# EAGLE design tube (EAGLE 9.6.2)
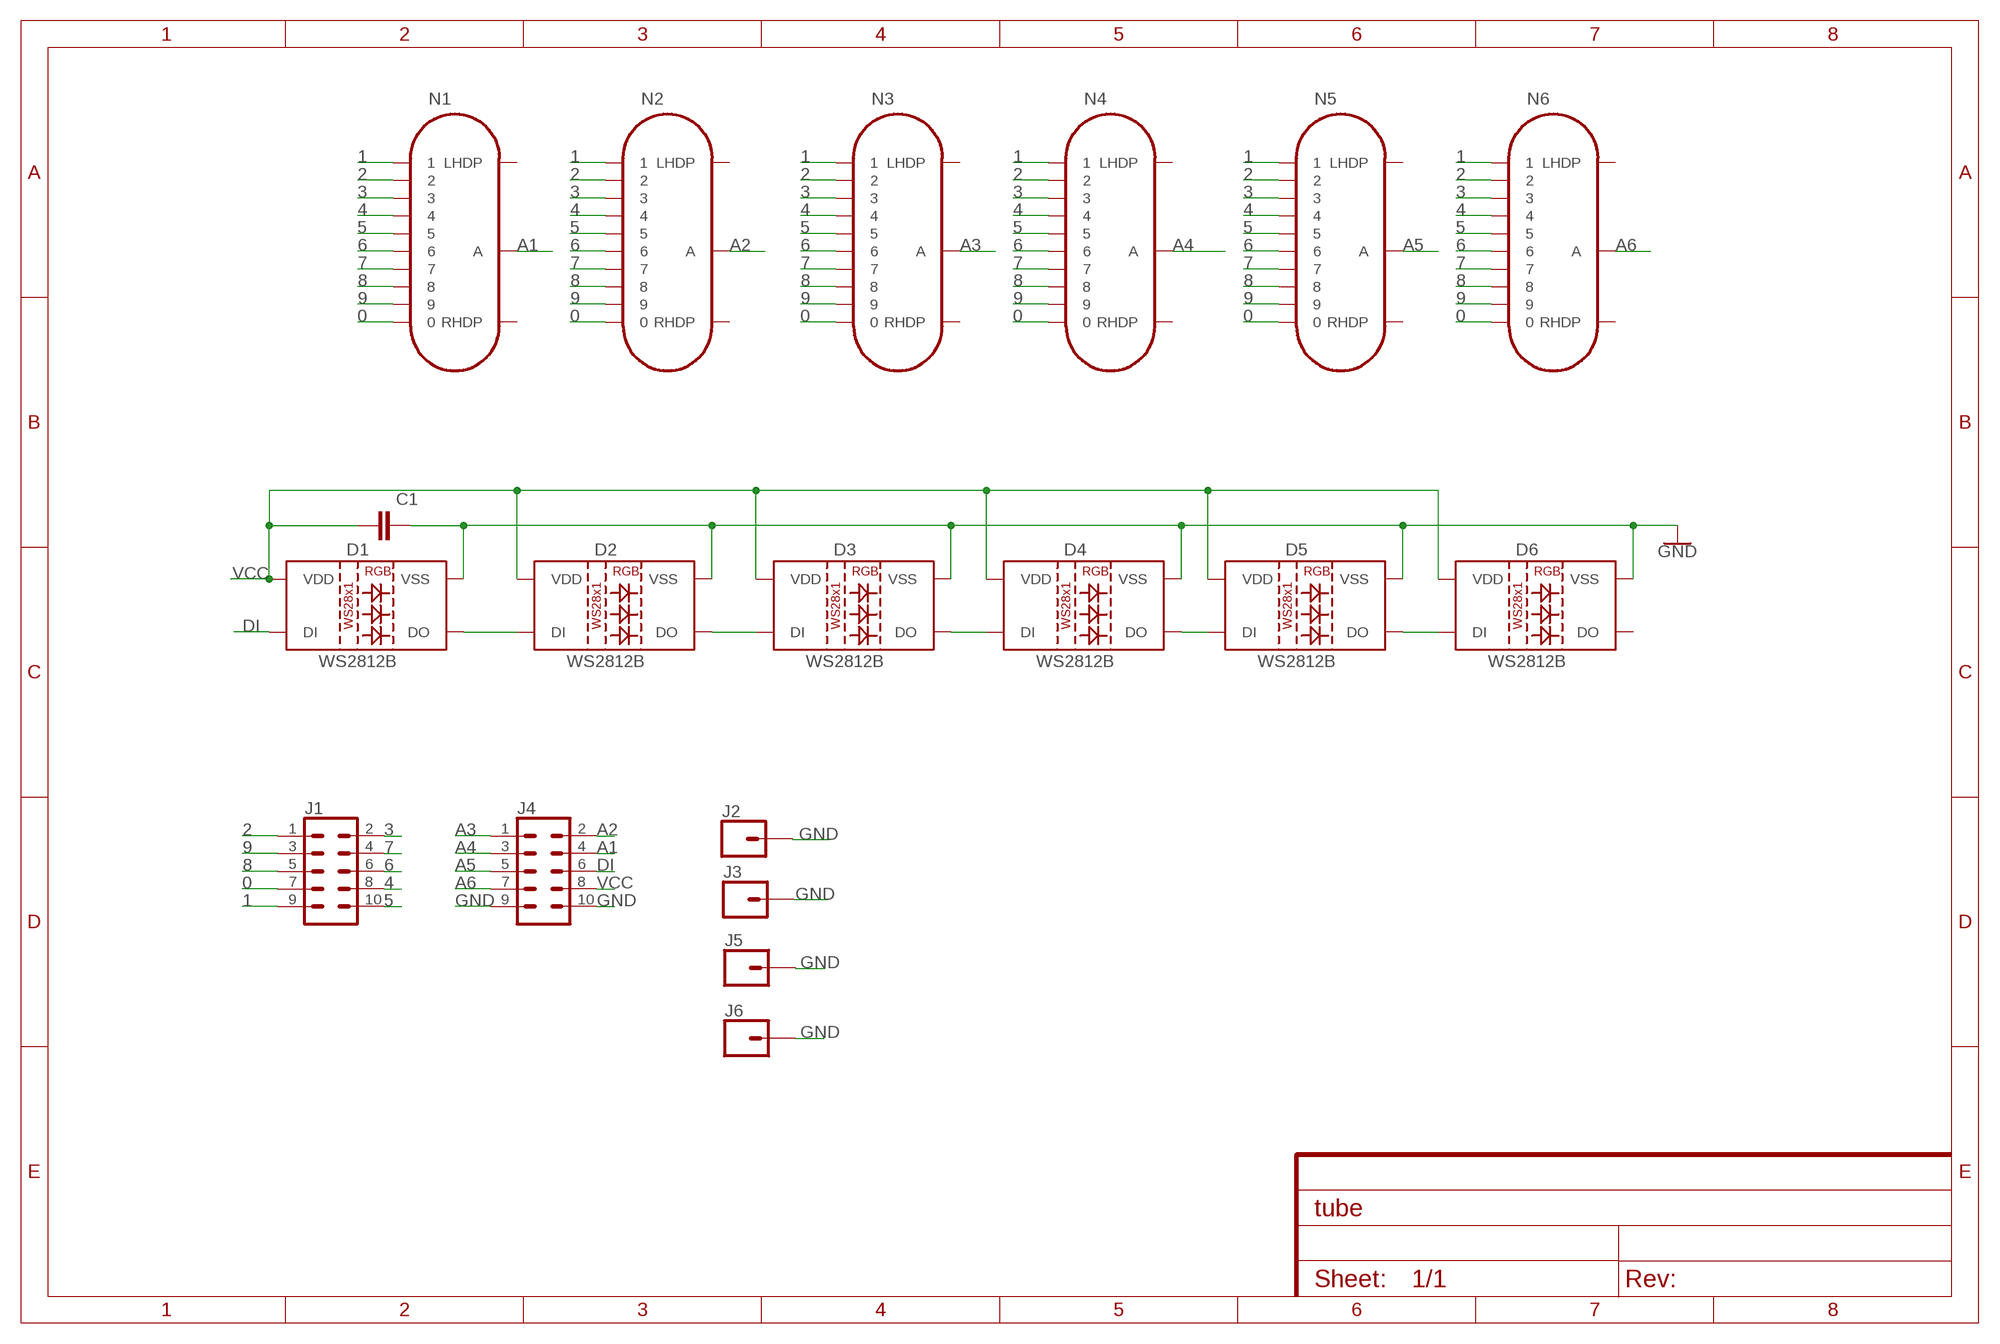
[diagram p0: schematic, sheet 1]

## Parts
C1  C-EUC1206  [C1206]
D1  WS2812B  [WS2812B]
D2  WS2812B  [WS2812B]
D3  WS2812B  [WS2812B]
D4  WS2812B  [WS2812B]
D5  WS2812B  [WS2812B]
D6  WS2812B  [WS2812B]
J1  CONN_05X2NO_SILK  [2X5_NOSILK]
J2  CONN_01PTH_2MM  [1X01_2MM]
J3  CONN_01PTH_2MM  [1X01_2MM]
J4  CONN_05X2NO_SILK  [2X5_NOSILK]
J5  CONN_01PTH_2MM  [1X01_2MM]
J6  CONN_01PTH_2MM  [1X01_2MM]
N1  IN-14  [IN-14]
N2  IN-14  [IN-14]
N3  IN-14  [IN-14]
N4  IN-14  [IN-14]
N5  IN-14  [IN-14]
N6  IN-14  [IN-14]

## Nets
0: J1.7 N1.0 N2.0 N3.0 N4.0 N5.0 N6.0
1: J1.9 N1.1 N2.1 N3.1 N4.1 N5.1 N6.1
2: J1.1 N1.2 N2.2 N3.2 N4.2 N5.2 N6.2
3: J1.2 N1.3 N2.3 N3.3 N4.3 N5.3 N6.3
4: J1.8 N1.4 N2.4 N3.4 N4.4 N5.4 N6.4
5: J1.10 N1.5 N2.5 N3.5 N4.5 N5.5 N6.5
6: J1.6 N1.6 N2.6 N3.6 N4.6 N5.6 N6.6
7: J1.4 N1.7 N2.7 N3.7 N4.7 N5.7 N6.7
8: J1.5 N1.8 N2.8 N3.8 N4.8 N5.8 N6.8
9: J1.3 N1.9 N2.9 N3.9 N4.9 N5.9 N6.9
A1: J4.4 N1.A
A2: J4.2 N2.A
A3: J4.1 N3.A
A4: J4.3 N4.A
A5: J4.5 N5.A
A6: J4.7 N6.A
DI: D1.4(DI) J4.6
GND: C1.2 D1.3(VSS) D2.3(VSS) D3.3(VSS) D4.3(VSS) D5.3(VSS) D6.3(VSS) J2.1 J3.1 J4.9 J4.10 J5.1 J6.1
N$1: D1.2(DO) D2.4(DI)
N$2: D2.2(DO) D3.4(DI)
N$3: D3.2(DO) D4.4(DI)
N$4: D4.2(DO) D5.4(DI)
N$5: D5.2(DO) D6.4(DI)
VCC: C1.1 D1.1(VDD) D2.1(VDD) D3.1(VDD) D4.1(VDD) D5.1(VDD) D6.1(VDD) J4.8
Unconnected: D6.2(DO) N1.LHDP N1.RHDP N2.LHDP N2.RHDP N3.LHDP N3.RHDP N4.LHDP N4.RHDP N5.LHDP N5.RHDP N6.LHDP N6.RHDP

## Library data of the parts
C1 = rcl:C-EU: CAPACITOR, European symbol; SPICEPREFIX: C
D1-D6 = SparkFun-LED:WS2812B: WS2812B SMD addressable RGB LED 5x5mm SMD LED with built-in controller IC. Color: Red/Green/Blue mC Rating: RGB: 390, 660, 180 mcd Forward Voltage: RGB: 2.0, 3.0, 3.0 V Packages:WS2812B SparkFun Products: Blynk Board - ESP8266; PROD_ID: DIO-12503
J1 J4 = SparkFun-Connectors:CONN_05X2: Multi connection point. Often used as Generic Header-pin footprint for 0.1 inch spaced/style header connections For AVR SPI programming port, see special device with nice symbol: "AVR_SPI_PROG_5x2.dev" You can populate with any combo of single row headers, but if you'd like an exact match, check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
J2 J3 J5 J6 = SparkFun-Connectors:CONN_01: Single connection point. Often used as Generic Header-pin footprint for 0.1 inch spaced/style header connections
N1-N6 = russian-nixies:IN-14: IN-14: medium numeric frontview nixie tube

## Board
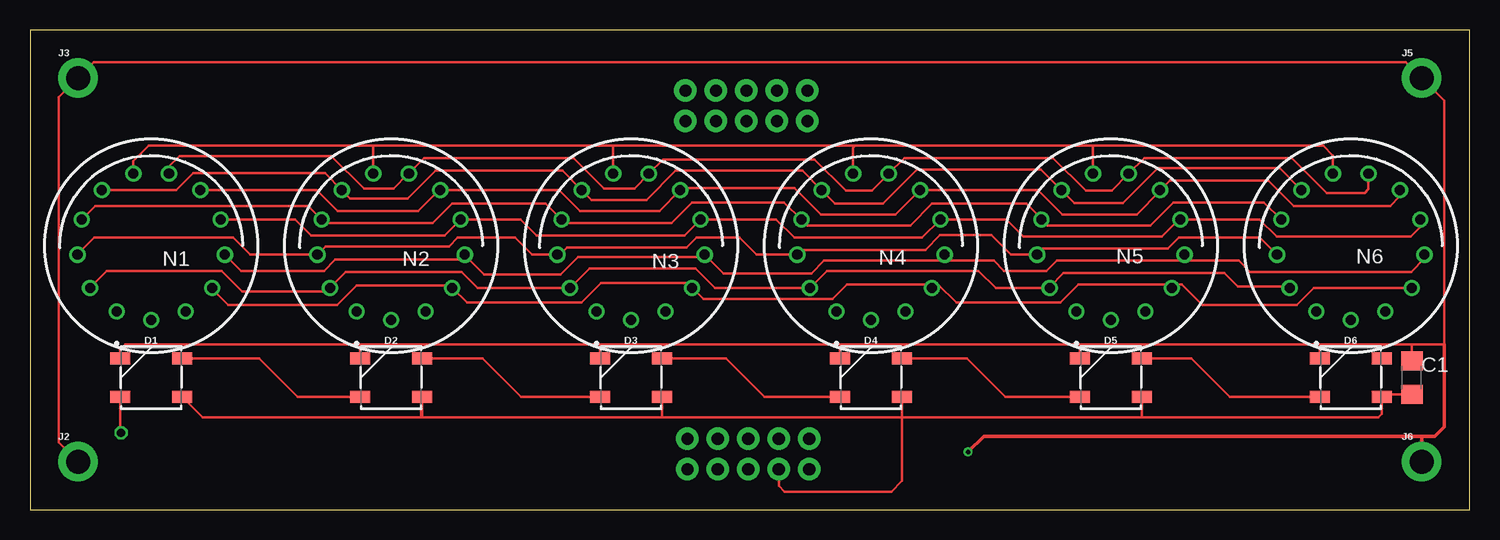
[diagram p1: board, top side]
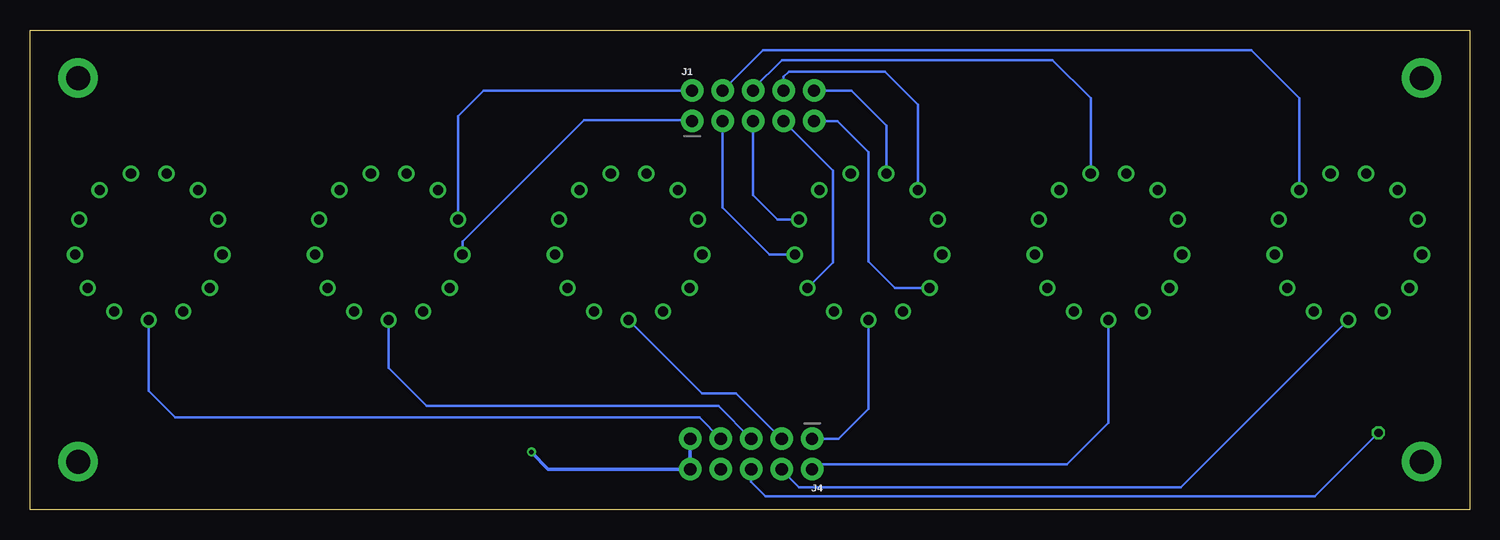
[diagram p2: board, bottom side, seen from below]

Size 120 x 40 mm. Coordinates in mm from the lower left corner, seen from the top.
Outline: 0,40 0,0 120,0 120,40 0,40
Copper layers (1*16): Top 0.035mm / dielectric 1.5mm / Bottom 0.035mm
Design rules "default": minimum track width 6mil, minimum drill 0.35mm, track to track 6mil, track to pad 6mil, pad to pad 6mil, via to via 6mil, smd to smd 6mil, copper to edge 40mil, drill to drill 6mil, minimum pad ring 10mil, minimum via ring 8mil, stop-mask expansion 4mil, vias tented up to drill 0mil, thermal gap 10mil

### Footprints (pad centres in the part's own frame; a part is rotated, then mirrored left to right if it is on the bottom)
C1206 = smd 1.6 x 1.8: 1 -1.4,0; 2 1.4,0
WS2812B = smd 1.651 x 1: 1 2.577,-1.6; 2 2.577,1.6; 3 -2.577,1.6; 4 -2.577,-1.6
2X5_NOSILK = drill 1.016 pad 1.88: 1 0,0; 2 0,2.54; 3 2.54,0; 4 2.54,2.54; 5 5.08,0; 6 5.08,2.54; 7 7.62,0; 8 7.62,2.54; 9 10.16,0; 10 10.16,2.54
1X01_2MM = drill 2 pad 3.302: 1 0,0
IN-14 = drill 0.84: 0 5.094,-3.516; 1 -5.094,-3.516; 2 -6.145,-0.746; 3 -5.788,2.195; 4 -4.105,4.633; 5 -1.481,6.01; 6 1.481,6.01; 7 4.105,4.633; 8 5.788,2.195; 9 6.145,-0.746; A 0,-6.19; LHDP 2.877,-5.481; RHDP -2.877,-5.481

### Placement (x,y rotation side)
C1  115.2,11 90 top
D1  10.1,11 0 top
D2  30.1,11 0 top
D3  50.1,11 0 top
D4  70.1,11 0 top
D5  90.1,11 0 top
D6  110.1,11 0 top
J1  64.8,32.4 0 bottom
J2  4,4 0 top
J3  4,36 0 top
J4  54.8,5.9 180 bottom
J5  116,36 0 top
J6  116,4 0 top
N1  10.1,22 0 top
N2  30.1,22 0 top
N3  50.1,22 0 top
N4  70.1,22 0 top
N5  90.1,22 0 top
N6  110.1,22 0 top

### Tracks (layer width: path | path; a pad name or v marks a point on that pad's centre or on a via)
0
  Top 0.2: N1.0 15.19,18.39 16.53,17.06 25.59,17.06 27.22,18.68 34.99,18.68 N2.0 35.21,18.48 36.43,17.26 45.99,17.26 47.62,18.88 54.79,18.88 N3.0 55.21,18.48 56.13,17.56 66.89,17.56 68.12,18.78 75.19,18.78 | 75.19,18.78 75.71,18.78 77.23,17.26 85.89,17.26 87.42,18.78 95.19,18.78 N5.0 95.19,18.68 95.29,18.78 96.01,18.78 97.73,17.06 105.59,17.06 107.02,18.48 N6.0 | N4.0 75.19,18.78
  Bottom 0.2: J1.7 53.06,28.28 53.06,20.61 N3.0
1
  Top 0.2: N1.1 5.01,18.5 6.41,19.91 15.98,19.91 17.71,18.18 24.71,18.18 N2.1 25.01,18.51 26.31,19.81 35.98,19.81 37.3,18.48 N3.1 46.64,20.11 55.48,20.11 57.1,18.48 N4.1 66.44,19.91 79.08,19.91 80.5,18.48 N5.1 85.01,18.57 86.14,19.71 99.58,19.71 100.7,18.58 104.91,18.58 N6.1
  Bottom 0.2: J1.9 52.7,32.4 50.1,29.8 50.1,20.7 47.88,18.48 N3.1
2
  Top 0.2: N1.2 3.96,21.27 5.36,22.68 16.93,22.68 18.36,21.25 N2.2 24.66,21.95 34.94,21.95 35.66,22.68 40.43,22.68 41.85,21.25 N3.2 44.16,21.25 44.76,21.85 54.73,21.85 55.56,22.68 59.13,22.68 60.55,21.25 N4.2 64.36,21.65 74.64,21.65 75.86,22.88 80.13,22.88 81.75,21.25 N5.2 84.45,21.75 94.83,21.75 95.76,22.68 102.53,22.68 N6.2 | N6.2
  Bottom 0.2: J1.1 64.9,32.5 73.81,32.5 83.95,22.35 N5.2
3
  Top 0.2: N1.3 5.44,25.32 23.19,25.32 N2.3 24.61,23.89 33.58,23.89 35.2,25.52 42.97,25.52 44.3,24.2 N3.3 44.61,23.89 53.48,23.89 55.2,25.62 62.87,25.62 64.3,24.2 N4.3 64.81,23.7 73.38,23.7 75.2,25.52 83.07,25.52 84.31,24.28 N5.3 84.81,23.7 93.38,23.7 95.3,25.62 102.87,25.62 104.3,24.2 N6.3
  Bottom 0.2: J1.2 82.17,34.94 84.31,32.8 N5.3
4
  Top 0.2: N1.4 12.2,26.63 13.62,28.06 24.59,28.06 26,26.65 N2.4 26.7,25.93 31.5,25.93 33.82,28.26 44.39,28.26 45.99,26.65 N3.4 46.8,25.83 51.39,25.83 53.82,28.26 64.39,28.26 66,26.65 N4.4 67.1,25.53 71.09,25.53 73.92,28.36 84.29,28.36 86,26.65 N5.4 87.08,25.55 91.11,25.55 94.02,28.46 104.19,28.46 106,26.65 N6.4
  Bottom 0.2: N4.4 66,26.65 | J1.8 57.18,36.09 56.73,36.53 48.75,36.53 45.99,33.78 N3.4
5
  Top 0.2: N1.5 8.62,29.06 9.9,30.34 28.6,30.34 | 28.6,30.34 48.62,30.34 | 68.8,30.34 88.7,30.34 | N2.5 28.6,28.03 28.6,30.34 | N3.5 48.62,30.34 | N4.5 68.62,30.16 68.8,30.34 | N5.5 88.62,30.25 88.7,30.34 | N6.5 108.62,29.51 107.79,30.34 88.7,30.34 | 48.62,30.34 68.8,30.34
  Bottom 0.2: J1.10 51.54,34.94 48.62,32.02 N3.5
6
  Top 0.2: N1.6 11.58,28.61 12.47,29.5 25.12,29.5 27.84,26.78 30.3,26.78 31.53,28.01 N2.6 32.87,29.3 45.32,29.3 47.84,26.78 50.4,26.78 51.58,27.96 N3.6 52.77,29.2 65.4,29.2 68.02,26.58 70.2,26.58 71.58,27.96 N4.6 72.88,29.31 85.29,29.31 88,26.6 90.17,26.6 N5.6 92.88,29.31 105.19,29.31 108.1,26.4 111.27,26.4 111.58,26.71 N6.6
  Bottom 0.2: J1.6 59.72,35.09 57.32,37.48 34.76,37.48 31.58,34.31 N2.6
7
  Top 0.2: N1.7 23.92,26.63 25.64,24.91 32.37,24.91 34.09,26.63 N2.7 44.12,26.63 45.84,24.91 52.47,24.91 N3.7 54.41,26.83 63.72,26.83 65.94,24.61 72.17,24.61 N4.7 84.02,26.63 86.04,24.61 92.27,24.61 94.2,26.55 N5.7 95,27.43 103.22,27.43 105.34,25.31 113.38,25.31 114.2,26.14 N6.7
  Bottom 0.2: J1.4 58.9,38.3 18.17,38.3 14.21,34.33 N1.7
8
  Top 0.2: N1.8 22.1,24.2 23.43,22.87 34.55,22.87 35.88,24.2 N2.8 40.9,24.2 42.23,22.87 54.55,22.87 55.88,24.2 N3.8 62.2,24.2 63.73,22.67 74.35,22.67 75.88,24.2 N4.8 81.4,24.2 82.83,22.77 94.35,22.77 95.78,24.2 N5.8 102.5,24.2 103.93,22.77 115.1,22.77 115.89,23.56 N6.8
  Bottom 0.2: J1.5 59.72,26.23 57.69,24.2 N3.8
9
  Top 0.2: N3.9 | N4.9 76.25,20.75 | N5.9 | N5.9 96.25,20.75 100.76,20.75 101.68,19.83 115.14,19.83 116.25,20.93 N6.9 | N2.9 36.24,20.85 | 36.24,20.85 36.6,20.85 37.85,19.6 44.24,19.6 45.69,21.05 56.04,21.05 N3.9 | 36.24,20.85 25.45,20.85 24.5,19.9 17.6,19.9 N1.9 | 76.25,20.75 80.34,20.75 81.2,19.9 84.74,19.9 85.59,20.75 96.25,20.75 N5.9 | 76.25,20.75 66.19,20.75 65.14,19.7 57.8,19.7 N3.9
  Bottom 0.2: J1.3 62.26,25.17 58.34,21.25 N3.9
A1
  Bottom 0.2: J4.4 57.34,3.31 55.89,1.87 24.04,1.87 N1.A
A2
  Bottom 0.2: J4.2 54.4,3.76 33.55,3.76 30.1,7.21 N2.A
A3
  Bottom 0.2: J4.1 52.6,5.9 50.1,8.4 N3.A
A4
  Bottom 0.2: J4.3 61.13,9.69 63.98,9.69 N4.A
A5
  Bottom 0.2: J4.5 62.62,8.64 86.93,8.64 90.1,11.81 N5.A
A6
  Bottom 0.2: J4.7 64.21,7.69 107.9,7.69 110.1,9.89 N6.A
DI  (via drill 0.7)
  Top 0.2: v7.6,6.4 7.52,6.48 D1.4
  Bottom 0.2: J4.6 59.88,2.31 58.68,1.12 12.88,1.12 v7.6,6.4
GND  (via drill 0.35)
  Top 0.2: D1.3 7.52,13.33 7.95,13.75 27.6,13.75 | 27.6,13.75 47.6,13.75 | 47.6,13.75 67.7,13.75 | 67.7,13.75 87.6,13.75 | 87.6,13.75 107.55,13.75 | 107.55,13.75 107.52,13.72 D6.3 | D2.3 27.52,13.68 27.6,13.75 | D3.3 47.52,13.68 47.6,13.75 | D4.3 67.52,13.57 67.7,13.75 | D5.3 87.52,13.68 87.6,13.75 | C1.2 115.2,13.75 | 115.2,13.75 107.55,13.75 | J2.1 2.4,5.6 2.4,34.4 J3.1 5.33,37.33 114.67,37.33 J5.1 117.9,34.1 117.9,13.75 115.2,13.75
  Top 0.3: v78.2,4.8 79.5,6.1 116,6.1 | J6.1 116,6.1 | 117.9,13.75 117.9,6.9 117.1,6.1 116,6.1
  Bottom 0.3: J4.9 J4.10 76.8,3.36 78.2,4.76 v78.2,4.8
N$1
  Top 0.2: D1.2 19.12,12.6 22.32,9.4 D2.4
N$2
  Top 0.2: D2.2 37.72,12.6 40.92,9.4 D3.4
N$3
  Top 0.2: D3.2 58.02,12.6 61.22,9.4 D4.4
N$4
  Top 0.2: D4.2 78.12,12.6 81.32,9.4 D5.4
N$5
  Top 0.2: D5.2 96.82,12.6 100.02,9.4 D6.4
VCC
  Top 0.2: D1.1 14.38,7.7 32.68,7.7 D2.1 32.6,9.32 32.6,7.7 52.68,7.7 | 52.68,7.7 D3.1 52.38,9.7 52.4,9.7 | D5.1 92.68,7.7 | 72.68,7.7 D4.1 72.68,9.57 72.55,9.7 72.5,9.7 | 92.68,7.7 72.68,7.7 | 92.68,7.7 112.38,7.7 112.68,8 D6.1 112.88,9.6 C1.1 | 72.68,7.7 52.68,7.7 | J4.8 62.42,1.96 62.88,1.5 71.8,1.5 72.68,2.38 72.68,7.7

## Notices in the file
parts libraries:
SparkFun-Aesthetics: Licensing: Creative Commons ShareAlike 4.0 International - https://creativecommons.org/licenses/by-sa/4.0
